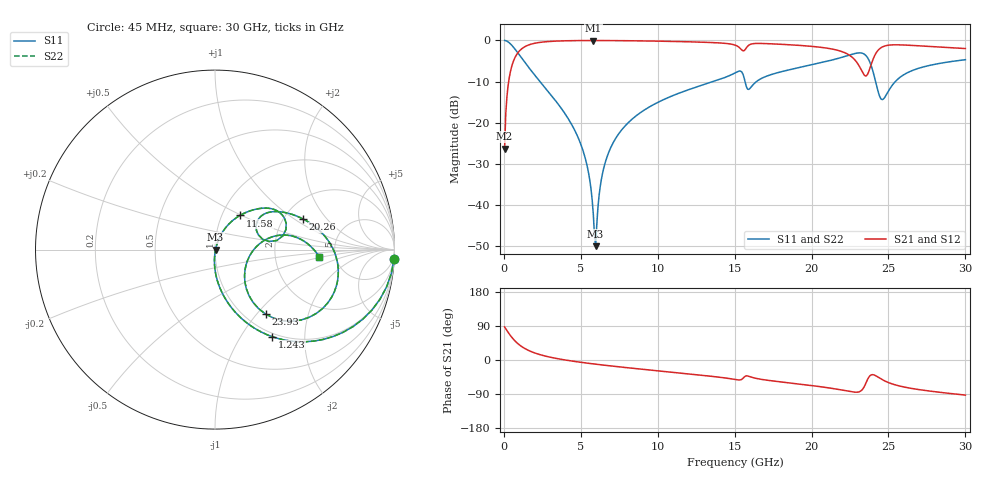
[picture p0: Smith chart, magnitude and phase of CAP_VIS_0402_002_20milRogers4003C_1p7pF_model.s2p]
! S-parameter model data by Modelithics Inc.  support@modelithics.com  813-866-6335  Tampa FL USA
! S-Parameter data specifications:
! Substrate: 20-mil Rogers 4003C, substrate thickness, H=0.508mm, Dielectric constant, Er=3.75
! PCB Mounting Pad Footprint: Pad width, PadW=0.50mm , Pad length, PadL=0.50mm , Pad gap, PadG (edge-to-edge)=0.40mm , Reference planes=1.4mm apart
! Created Wed Nov 18 12:42:58 2015
# hz S ma R 50
! 2 Port Network Data from SP1.SP block
! freq  magS11  angS11  magS21  angS21  magS12  angS12  magS22  angS22
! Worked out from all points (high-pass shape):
!   401 points, 45 MHz to 30 GHz, reference 50 ohm
!   highest |S21| = -0.03 dB at 5.811 GHz (marker M1); lowest = -26.3 dB at 45 MHz (marker M2)
!   |S21| within 3 dB of the highest: 903.4 MHz to 22.18 GHz (21.28 GHz wide, 184 % of centre); 24.2 GHz to end of sweep
!   lowest |S11| = -50.0 dB at 5.961 GHz (marker M3), VSWR 1.01, Z = 50.3 + j0.0314 ohm
!   |S11| at or under -10 dB: 2.346 GHz to 13.6 GHz (11.25 GHz wide, 141 % of centre); 15.67 GHz to 16.42 GHz (741.8 MHz wide, 4.62 % of centre); 24.16 GHz to 25.44 GHz (1.28 GHz wide, 5.16 % of centre)
!   |S22| runs from -50.0 to 0.0 dB; largest |S21 - S12| = 0
!   S11 on the Smith chart (normalised r, x): 45 MHz: 1, -40; 1.243 GHz: 0.95, -1.38; 11.58 GHz: 1.21, +0.49; 20.26 GHz: 2.52, +1.18; 23.93 GHz: 1.23, -1.12; 30 GHz: 3.74, -0.47
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4.5e7  0.9988 -2.9  0.04858 87.1  0.04858 87.1  0.9988 -2.9
4.194375e8  0.9099 -25.3  0.4145 64.7  0.4145 64.7  0.9099 -25.3
1.2432e9  0.5796 -56.8  0.8137 33.1  0.8137 33.1  0.5796 -56.8
2.516288e9  0.2894 -77.4  0.9553 12.2  0.9553 12.2  0.2894 -77.4
5.062462e9  0.05081 -93.3  0.9958 -6.4  0.9958 -6.4  0.05081 -93.3
5.511788e9  0.02404 -91.8  0.9966 -8.8  0.9966 -8.8  0.02404 -91.8
5.811338e9  0.007747 -77.6  0.9968 -10.3  0.9968 -10.3  0.007747 -77.6
5.961112e9  0.003169 5.7  0.9968 -11.0  0.9968 -11.0  0.003169 5.7
6.410438e9  0.02423 69.3  0.9964 -13.2  0.9964 -13.2  0.02423 69.3
7.084425e9  0.05637 70.3  0.9949 -16.3  0.9949 -16.3  0.05637 70.3
1.007992e10  0.1796 59.7  0.9792 -28.9  0.9792 -28.9  0.1796 59.7
1.157768e10  0.236 53.8  0.9665 -35.0  0.9665 -35.0  0.236 53.8
1.50225e10  0.4027 33.2  0.8775 -51.4  0.8775 -51.4  0.4027 33.2
1.592115e10  0.2542 24.6  0.8743 -43.0  0.8743 -43.0  0.2542 24.6
2.003996e10  0.5071 20.6  0.8457 -67.6  0.8457 -67.6  0.5071 20.6
2.026462e10  0.5181 19.3  0.8378 -68.8  0.8378 -68.8  0.5181 19.3
2.303546e10  0.7046 -14.2  0.5102 -84.5  0.5102 -84.5  0.7046 -14.2
2.355968e10  0.6466 -35.7  0.3712 -58.5  0.3712 -58.5  0.6466 -35.7
2.393411e10  0.4569 -51.9  0.5489 -38.7  0.5489 -38.7  0.4569 -51.9
2.453321e10  0.193 -26.5  0.8195 -50.3  0.8195 -50.3  0.193 -26.5
2.505742e10  0.2532 7.8  0.8776 -60.5  0.8776 -60.5  0.2532 7.8
3e10  0.5833 -4.1  0.7964 -92.6  0.7964 -92.6  0.5833 -4.1
